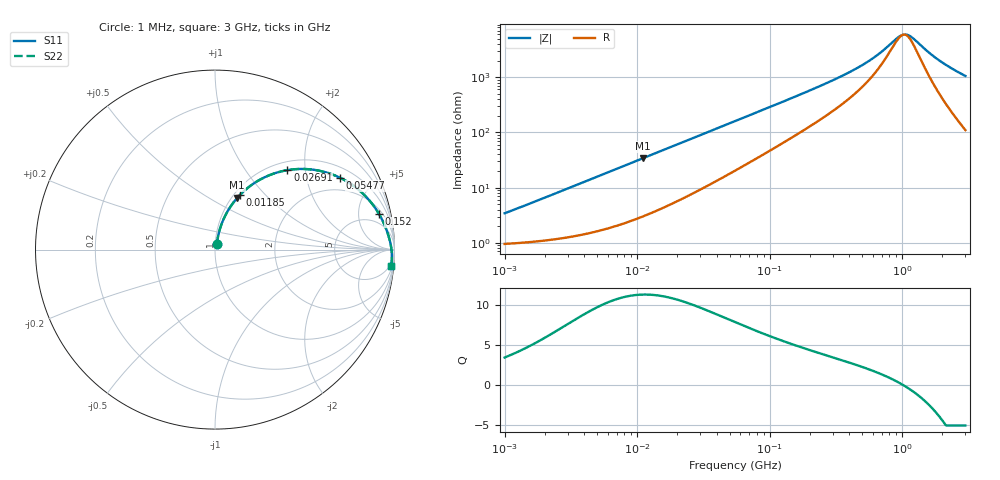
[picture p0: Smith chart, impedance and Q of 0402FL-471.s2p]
# MHz S MA R 50
!Freq  MagS11  AngS11  MagS21  AngS21  MagS12  AngS12  MagS22  AngS22
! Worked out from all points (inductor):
!   801 points, 1 MHz to 3 GHz, reference 50 ohm
!   read as one part in series: L = 521 nH near 1.041 MHz
!   highest Q = 11.3 at 11.04 MHz (marker M1), where L = 489 nH
!   self-resonance near 1.023 GHz
!   S11 on the Smith chart (normalised r, x): 1 MHz: 1.02, +0.07; 11.85 MHz: 1.06, +0.73; 26.91 MHz: 1.16, +1.60; 54.77 MHz: 1.41, +3.18; 152 MHz: 2.70, +8.52; 3 GHz: 3, -21
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1  0.03402 71.9  0.99 -1.9  0.99 -1.9  0.03402 71.9
3.823119  0.1196 76.6  0.9792 -6.8  0.9792 -6.8  0.1196 76.6
6.969505  0.2092 72.6  0.9586 -12.0  0.9586 -12.0  0.2092 72.6
11.04425  0.3141 66.7  0.922 -18.2  0.922 -18.2  0.3141 66.7
11.84571  0.3331 65.5  0.9139 -19.4  0.9139 -19.4  0.3331 65.5
14.47069  0.3919 61.9  0.8857 -23.0  0.8857 -23.0  0.3919 61.9
26.91325  0.599 47.7  0.743 -36.6  0.743 -36.6  0.599 47.7
37.82194  0.7081 38.9  0.6319 -44.7  0.6319 -44.7  0.7081 38.9
54.77226  0.804 29.8  0.5015 -52.9  0.5015 -52.9  0.804 29.8
88.54986  0.8862 20.0  0.3468 -61.1  0.3468 -61.1  0.8862 20.0
152.0175  0.9355 12.2  0.2153 -66.6  0.2153 -66.6  0.9355 12.2
209.4008  0.9519 8.9  0.1584 -67.9  0.1584 -67.9  0.9519 8.9
331.8279  0.9667 5.4  0.09792 -67.4  0.09792 -67.4  0.9667 5.4
471.0174  0.9739 3.4  0.06385 -64.1  0.06385 -64.1  0.9739 3.4
623.3561  0.9781 2.1  0.04177 -57.3  0.04177 -57.3  0.9781 2.1
792.5923  0.9809 1.0  0.02617 -42.8  0.02617 -42.8  0.9809 1.0
977.9672  0.983 0.2  0.01733 -10.4  0.01733 -10.4  0.983 0.2
1048.936  0.9835 -0.1  0.01655 6.1  0.01655 6.1  0.9835 -0.1
1113.852  0.984 -0.3  0.01708 20.4  0.01708 20.4  0.984 -0.3
1206.698  0.9846 -0.7  0.01937 36.9  0.01937 36.9  0.9846 -0.7
1874.306  0.9866 -2.6  0.0477 72.4  0.0477 72.4  0.9866 -2.6
3000  0.9858 -5.3  0.09364 78.6  0.09364 78.6  0.9858 -5.3
